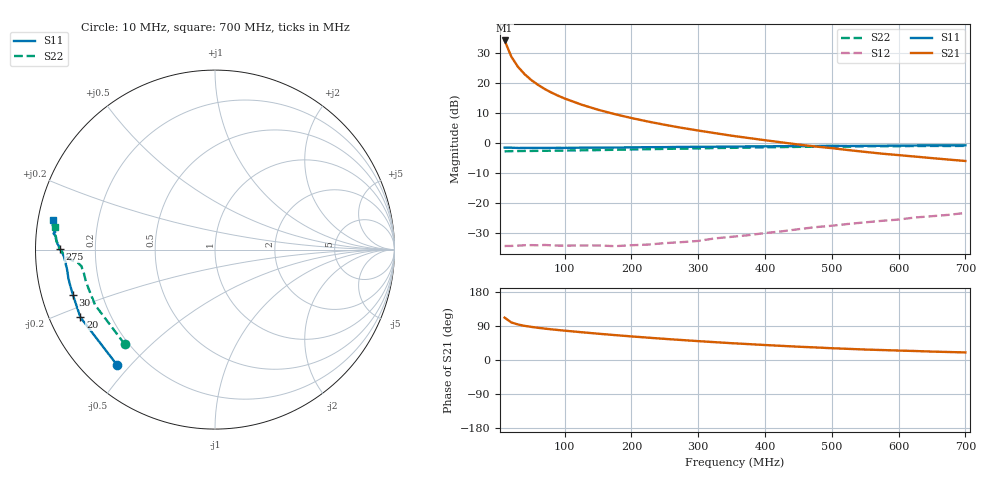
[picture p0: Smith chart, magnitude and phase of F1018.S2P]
! Date: Fri Aug 11 10:19:49 1995
# MHZ  S  MA  R  50.0000
!  POLYFET RF DEVICES
!  F1018 (Each Side)
!  S PARAMETERS
!  VDS=28V, IDQ=600mA
!FREQ  S11MAG S11ANG S21MAG S21ANG S12MAG S12ANG S22MAG S22ANG
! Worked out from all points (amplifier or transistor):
!   34 points, 10 MHz to 700 MHz, reference 50 ohm
!   highest |S21| = 34.1 dB at 10 MHz (marker M1)
!   |S21| within 3 dB of that: start of sweep to 15.61 MHz
!   unconditionally stable (mu >= 1): 199.2 MHz to 400.2 MHz
!   at 60 MHz: K = 0.33, MSG = 26.6 dB, |S12| = -33.9 dB
!   at 300 MHz: K = 1.14, MAG = 16.0 dB, |S12| = -32.5 dB
!   at 700 MHz: K = 0.64, MSG = 8.6 dB, |S12| = -23.2 dB
!   S11 on the Smith chart (normalised r, x): 10 MHz: 0.10, -0.46; 20 MHz: 0.09, -0.24; 30 MHz: 0.09, -0.16; 275 MHz: 0.07, +0.00; 700 MHz: 0.04, +0.09
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10  0.8431 -130.3  50.6 111.8  0.01959 22.5  0.7289 -133.5
20  0.8395 -153.3  27.33 99.2  0.01965 15.2  0.7358 -155.2
30  0.8308 -162.1  18.46 93.7  0.01984 11.9  0.7373 -162.9
40  0.8315 -166.6  13.91 90.1  0.02017 10.4  0.7413 -166.8
50  0.8324 -169.3  11.12 87.4  0.02025 11.3  0.7414 -168.9
60  0.8311 -171.3  9.271 85.0  0.02015 10.9  0.7434 -170.6
70  0.832 -172.6  7.917 82.9  0.02037 12.2  0.7452 -171.5
80  0.8325 -173.5  6.911 81.0  0.02011 14.3  0.7481 -172.1
90  0.8359 -174.3  6.129 79.2  0.01989 13.9  0.7491 -172.9
100  0.8339 -174.9  5.497 77.4  0.01984 15.0  0.7517 -173.1
125  0.8395 -176.1  4.356 73.3  0.02002 19.9  0.7594 -173.8
150  0.842 -177.1  3.58 69.4  0.02002 21.8  0.7655 -174.4
175  0.8448 -177.9  3.026 65.8  0.01946 27.0  0.775 -174.7
200  0.8496 -178.5  2.607 62.2  0.02017 30.2  0.7836 -175.2
225  0.856 -179.2  2.278 58.9  0.0207 34.9  0.7921 -175.5
250  0.8579 -179.8  2.011 55.8  0.02186 39.7  0.8017 -175.8
275  0.8659 179.7  1.794 52.7  0.02269 44.5  0.8109 -176.2
325  0.8711 178.6  1.464 47.0  0.02622 52.7  0.8287 -177.3
375  0.8809 177.5  1.217 42.0  0.02962 57.7  0.8441 -178.4
475  0.8943 175.0  0.8792 33.2  0.04021 63.9  0.8693 179.0
600  0.9088 172.0  0.6316 24.9  0.05385 66.1  0.8897 175.4
700  0.9172 169.7  0.5053 19.9  0.06933 65.2  0.8993 172.1
